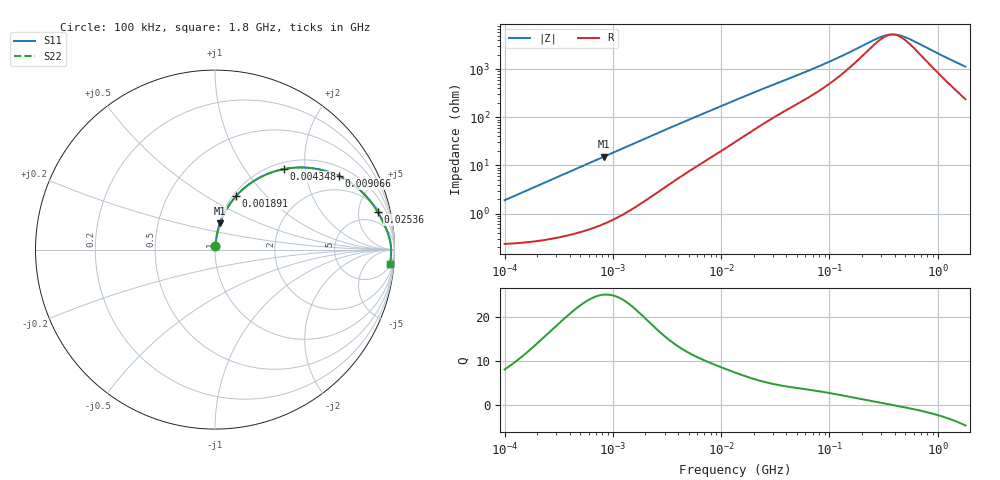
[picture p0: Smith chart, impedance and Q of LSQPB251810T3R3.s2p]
! LSQPB251810T3R3  S-PARAMETER MODEL  ( General Type )
! Model Generated by TAIYO YUDEN Corporation (http://www.ty-top.com)
! Version 2.0
! TAIYO YUDEN Control No. 100810NG22EB-FKC
! Copyright(c) 2009 TAIYO YUDEN CO.,LTD. All Rights Reserved.
! Product Description (link to TY-COMPAS)
! https://ds.yuden.co.jp/TYCOMPAS/or/detail?pn=LSQPB251810T3R3M&u=M
! Products Name : Inductors
! Characteristics :
!  Inductance : 3.3 uH , SRF(min) : 70 MHz , DC Resistance(max) : 0.286 Ohm
!  Rated Current : Saturation :700 mA , Temp Rise : 700 mA (40 degC)
!  Case Size : 2.5 x 1.8 / 0.098 x 0.071 [mm/inch] , Thickness : 1.0 / 0.04 [mm/inch]
!  (Conditions: Temperature = 25 degC , DC Bias Current/Voltage = 0A / 0V)
! External Node Assignments :
!  1  o---GGG---o  2
! GND o---------o GND
! Frequency Range : 0.1MHz  -  1800MHz  [ 402 STEP ]
# MHz S RI R 50
! Freq[MHz].  S11 Real  S11 Imag  S21 Real  S21 Imag  S12 Real  S12 Imag  S22 Real  S22 Imag
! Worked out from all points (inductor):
!   401 points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, 100 kHz to 1.8 GHz, reference 50 ohm
!   read as one part in series: L = 2.98 uH near 105 kHz
!   highest Q = 25 at 822 kHz (marker M1), where L = 2.94 uH
!   self-resonance near 380.1 MHz
!   S11 on the Smith chart (normalised r, x): 100 kHz: 1.00, +0.04; 1.891 MHz: 1.03, +0.69; 4.348 MHz: 1.12, +1.55; 9.066 MHz: 1.35, +3.10; 25.36 MHz: 2.54, +7.98; 1.8 GHz: 6, -22
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0.1  0.00268 0.0187  0.9973 -0.0187  0.9973 -0.0187  0.00268 0.0187
0.253659  0.00511 0.047  0.9949 -0.047  0.9949 -0.047  0.00511 0.047
0.516129  0.0131 0.094  0.9869 -0.094  0.9869 -0.094  0.0131 0.094
0.822022  0.0281 0.1465  0.9719 -0.1465  0.9719 -0.1465  0.0281 0.1465
1.309209  0.0632 0.2229  0.9368 -0.2229  0.9368 -0.2229  0.0632 0.2229
1.890522  0.1184 0.2992  0.8816 -0.2992  0.8816 -0.2992  0.1184 0.2992
2.66389  0.2034 0.3737  0.7966 -0.3737  0.7966 -0.3737  0.2034 0.3737
4.347904  0.3846 0.4488  0.6154 -0.4488  0.6154 -0.4488  0.3846 0.4488
6.126528  0.5337 0.4545  0.4663 -0.4545  0.4663 -0.4545  0.5337 0.4545
9.066201  0.6901 0.41  0.3099 -0.41  0.3099 -0.41  0.6901 0.41
13.41641  0.8059 0.3333  0.1941 -0.3333  0.1941 -0.3333  0.8059 0.3333
18.00091  0.8637 0.2724  0.1363 -0.2724  0.1363 -0.2724  0.8637 0.2724
25.36465  0.9072 0.2095  0.0928 -0.2095  0.0928 -0.2095  0.9072 0.2095
69.24595  0.9639 0.0894  0.0361 -0.0894  0.0361 -0.0894  0.9639 0.0894
127.7465  0.976 0.0471  0.024 -0.0471  0.024 -0.0471  0.976 0.0471
272.9811  0.9808 0.0123  0.0192 -0.0123  0.0192 -0.0123  0.9808 0.0123
316.1998  0.9811 0.00678  0.0189 -0.00678  0.0189 -0.00678  0.9811 0.00678
357.3983  0.9813 0.00226  0.0187 -0.00226  0.0187 -0.00226  0.9813 0.00226
424.248  0.9814 -0.00405  0.0186 0.00405  0.0186 0.00405  0.9814 -0.00405
516.0898  0.9814 -0.0114  0.0186 0.0114  0.0186 0.0114  0.9814 -0.0114
1216.359  0.9789 -0.053  0.0211 0.053  0.0211 0.053  0.9789 -0.053
1800  0.9748 -0.0827  0.0252 0.0827  0.0252 0.0827  0.9748 -0.0827
